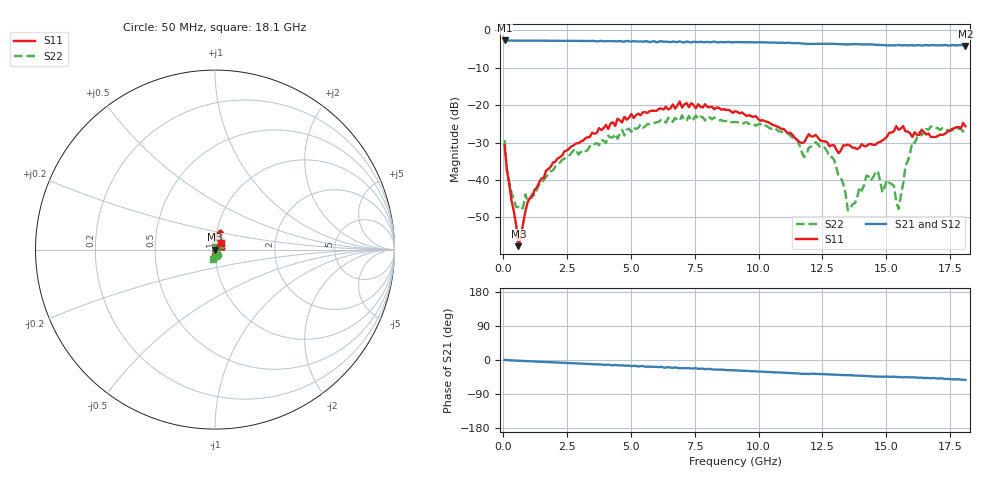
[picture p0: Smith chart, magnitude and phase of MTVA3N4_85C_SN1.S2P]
! Network Analyzer HP8720D.06.14 Serial No. US36140669
! 27 Jun 2005  09:42:14
! Frequency  S11  S21  S12  S22
# HZ  S  DB R 50
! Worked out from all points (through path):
!   201 points, 50 MHz to 18.1 GHz, reference 50 ohm
!   highest |S21| = -2.72 dB at 50 MHz (marker M1); lowest = -4.2 dB at 18.1 GHz (marker M2)
!   group delay of S21, straight-line fit = 7.99 ps
!   lowest |S11| = -57.7 dB at 591.5 MHz (marker M3), VSWR 1.00, Z = 50.1 - j0.0227 ohm
!   |S11| at or under -10 dB: start of sweep to end of sweep
!   |S22| runs from -48.1 to -22.7 dB; largest |S21 - S12| = 0.021
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5e7  -30.71 -79.2  -2.72 0.2  -2.74 0.4  -29.35 -71.2
1.4025e8  -37.38 -77.9  -2.78 -0.3  -2.77 -0.2  -37.35 -97.3
3.2075e8  -45.57 -71.0  -2.73 -0.8  -2.74 -0.8  -43.53 -117.3
5.915e8  -57.71 -10.0  -2.75 -1.7  -2.77 -1.8  -47.27 -166.7
9.525e8  -45.94 48.6  -2.78 -2.9  -2.76 -3.0  -45.59 150.6
1.6745e9  -37.50 52.8  -2.80 -5.3  -2.79 -5.3  -39.21 111.2
3.1185e9  -29.54 58.3  -2.85 -9.5  -2.87 -9.7  -31.98 96.0
6.09675e9  -20.97 67.5  -3.02 -18.7  -2.96 -18.7  -24.43 63.3
9.075e9  -21.65 83.0  -3.17 -27.3  -3.15 -27.4  -24.52 32.6
1.115075e10  -27.48 88.9  -3.31 -34.3  -3.37 -34.5  -27.55 17.5
1.17825e10  -29.96 103.1  -3.57 -36.5  -3.55 -36.7  -33.86 29.1
1.21435e10  -28.37 87.6  -3.66 -36.1  -3.63 -36.4  -30.81 47.1
1.295575e10  -30.71 62.4  -3.63 -38.9  -3.65 -39.0  -34.59 27.0
1.349725e10  -30.54 37.5  -3.77 -40.1  -3.76 -40.1  -48.09 0.7
1.421925e10  -31.01 1.8  -3.79 -42.0  -3.79 -42.2  -38.88 -119.7
1.46705e10  -30.04 1.9  -3.88 -43.9  -3.88 -43.9  -37.59 -137.9
1.4851e10  -29.44 8.0  -3.98 -44.3  -3.92 -44.1  -43.40 -143.2
1.512175e10  -27.38 10.7  -4.05 -44.3  -3.98 -44.2  -40.77 -113.0
1.548275e10  -26.58 10.8  -3.90 -44.9  -4.03 -44.9  -47.77 -50.2
1.57535e10  -27.02 3.4  -3.98 -45.1  -4.14 -45.7  -36.25 -18.5
1.6295e10  -27.97 15.1  -3.98 -46.6  -3.99 -47.9  -27.18 -43.8
1.81e10  -25.63 49.0  -4.17 -52.3  -4.13 -53.2  -25.80 -100.7
